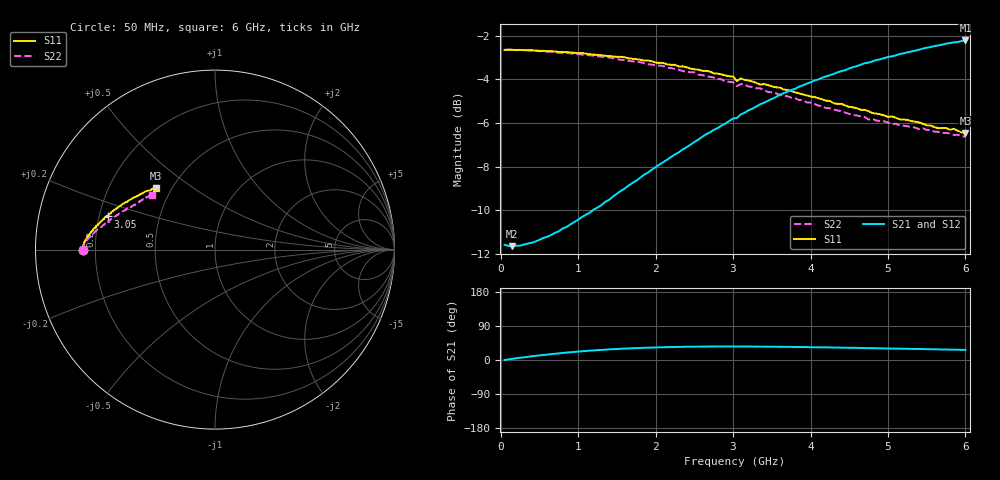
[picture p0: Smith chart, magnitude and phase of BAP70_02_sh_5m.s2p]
!	Created	by	janssen	on	Thu	Dec	12	13:21:33	MET	2002
#	HZ	S	MA	R	50
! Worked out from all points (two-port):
!   120 points, 50 MHz to 6 GHz, reference 50 ohm
!   highest |S21| = -2.21 dB at 6 GHz (marker M1); lowest = -11.7 dB at 150 MHz (marker M2)
!   |S21| within 3 dB of the highest: 3.317 GHz to end of sweep
!   lowest |S11| = -6.5 dB at 6 GHz (marker M3), VSWR 2.81, Z = 20.5 + j18.2 ohm
!   |S11| at or under -10 dB: nowhere
!   |S22| runs from -6.6 to -2.6 dB; largest |S21 - S12| = 0.015
!   S11 on the Smith chart (normalised r, x): 50 MHz: 0.15, -0.00; 3.05 GHz: 0.23, +0.14; 6 GHz: 0.41, +0.36
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5e7  0.7374 -179.8  0.2632 0.0  0.2625 -0.0  0.738 -179.8
1.5e8  0.738 179.6  0.2613 3.2  0.2611 3.1  0.738 179.5
5e8  0.7342 178.1  0.2703 12.1  0.2692 12.0  0.7329 178.3
7.5e8  0.7297 177.3  0.2827 17.5  0.2827 17.4  0.7274 177.3
1.05e9  0.7258 176.0  0.3049 23.0  0.3031 22.8  0.7193 176.2
1.6e9  0.7098 173.6  0.3543 30.2  0.3526 29.7  0.6993 173.9
2.05e9  0.6888 170.8  0.4024 33.4  0.3993 33.3  0.6789 171.9
2.35e9  0.6765 168.8  0.436 34.8  0.4319 34.6  0.6596 170.1
2.5e9  0.6659 168.2  0.4532 35.2  0.4494 35.0  0.6548 169.3
3e9  0.6409 163.9  0.5133 35.8  0.5068 35.5  0.6218 165.8
3.05e9  0.626 162.8  0.5147 35.5  0.5082 35.6  0.6092 165.4
3.1e9  0.634 163.2  0.5246 35.7  0.5181 35.7  0.6158 165.3
3.35e9  0.614 160.8  0.5534 35.2  0.5464 35.4  0.6019 163.1
3.6e9  0.6051 158.5  0.5814 34.9  0.572 35.1  0.5818 161.3
4.05e9  0.575 153.8  0.6271 33.6  0.6196 34.0  0.5544 157.2
4.3e9  0.5563 151.5  0.6498 32.9  0.6431 33.2  0.5383 154.5
4.35e9  0.5545 150.6  0.6553 32.8  0.6492 33.3  0.5354 154.8
4.4e9  0.5548 150.5  0.6595 32.6  0.6511 33.0  0.5335 154.2
4.55e9  0.5443 148.8  0.6732 32.3  0.6642 32.7  0.5226 152.8
5.05e9  0.5188 143.5  0.713 30.3  0.7068 31.0  0.4977 147.8
5.55e9  0.4946 138.1  0.7488 28.4  0.743 29.1  0.4826 142.8
6e9  0.4755 133.7  0.7754 26.7  0.7754 27.5  0.4661 139.2
